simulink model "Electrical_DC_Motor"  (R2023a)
settings: Solver=VariableStepAuto  StartTime=0.0  StopTime=10.0  RelTol=1e-3
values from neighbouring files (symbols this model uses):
  K = 1    [Electrical_DC_Motor_EQN.m]    (also in Electrical_DC_Motor_SLX_m.m; SI_Units.m)
undefined symbols (not defined in the file or in its folder): eTr
libraries: fl_lib x8, nesl_utility x1

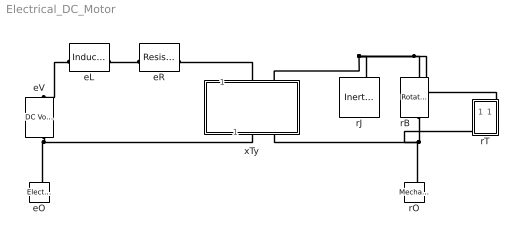
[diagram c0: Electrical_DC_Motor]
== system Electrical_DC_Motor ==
  eL : fl_lib/Electrical/Electrical Elements/Inductor  l=1e-6 H  r=0 Ohm  g=1e-9 1/Ohm  i_specify=off  i_priority=None  i=0 A  i_nominal_specify=off  i_nominal_unit=A  i_nominal_value=1  v_specify=off  v_priority=None  v=0 V  v_nominal_specify=off  v_nominal_unit=V  v_nominal_value=1  i_L_specify=off  i_L_priority=High  i_L=0 A  i_L_nominal_specify=off  i_L_nominal_unit=A  i_L_nominal_value=1
  eO : fl_lib/Electrical/Electrical Elements/Electrical Reference
  eR : fl_lib/Electrical/Electrical Elements/Resistor  R=1 Ohm  i_specify=off  i_priority=None  i=0 A  i_nominal_specify=off  i_nominal_unit=A  i_nominal_value=1  v_specify=off  v_priority=None  v=0 V  v_nominal_specify=off  v_nominal_unit=V  v_nominal_value=1
  eV : fl_lib/Electrical/Electrical Sources/DC Voltage Source  v0=1 V
  rB : fl_lib/Mechanical/Rotational Elements/Rotational Damper  D=0.001 N*m*s/rad  w_specify=off  w_priority=None  w=0 rad/s  w_nominal_specify=off  w_nominal_unit=rad/s  w_nominal_value=1  t_specify=off  t_priority=None  t=0 N*m  t_nominal_specify=off  t_nominal_unit=N*m  t_nominal_value=1
  rJ : fl_lib/Mechanical/Rotational Elements/Inertia  inertia=0.01 kg*m^2  num_ports=foundation.enum.numPorts2.one  w_specify=off  w_priority=High  w=0 rad/s  w_nominal_specify=off  w_nominal_unit=rad/s  w_nominal_value=1  t_specify=off  t_priority=None  t=0 N*m  t_nominal_specify=off  t_nominal_unit=N*m  t_nominal_value=1
  rO : fl_lib/Mechanical/Rotational Elements/Mechanical Rotational Reference
  rT : Subsystem  mask{rT='Ta'}
      mask prompts: rT "Output variable"
  xTy : Subsystem  mask{Transformer_type=eTr, T_type=F2=K*F1, xTy=K}
      mask prompts: Transformer_type "Type of Transformer"; T_type "Type of relation"; xTy "Name of parameter K"
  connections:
  eV/RConn1 -- xTy/RConn1 -- eO/LConn1
  eL/LConn1 -- eV/LConn1
  eR/LConn1 -- eL/RConn1
  xTy/LConn1 -- eR/RConn1
  rT/LConn1 -- rB/LConn1 -- xTy/LConn2 -- rJ/LConn1
  rB/RConn1 -- xTy/RConn2 -- rO/LConn1 -- rT/RConn1

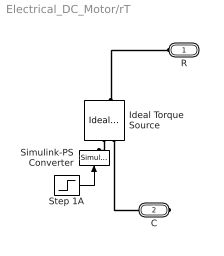
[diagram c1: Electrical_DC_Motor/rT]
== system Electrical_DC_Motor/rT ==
  Ideal Torque Source : fl_lib/Mechanical/Mechanical Sources/Ideal Torque Source
  Simulink-PS Converter : nesl_utility/Simulink-PS Converter  PhysicalDomain=network_engine_domain  SubClassName=ps_input  LeftPortType=input  RightPortType=output  PseudoPeriodic=off  Frequencies=[]  NoiseDistribution=none  NoiseParameters=[]  Unit=1  AffineConversion=off  FilteringAndDerivatives=zero  SimscapeFilterOrder=1  InputFilterTimeConstant=.001  UdotUserProvided=0
  Step 1A : Step  After=100  SampleTime=0
  R : PMIOPort  Side=Left
  C : PMIOPort  Port=2  Side=Right
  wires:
  Step 1A/1 -> Simulink-PS Converter/1
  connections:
  Ideal Torque Source/RConn2 -- C/RConn1
  Ideal Torque Source/LConn1 -- R/RConn1
  Ideal Torque Source/RConn1 -- Simulink-PS Converter/RConn1

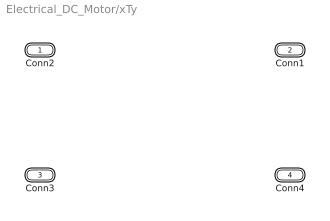
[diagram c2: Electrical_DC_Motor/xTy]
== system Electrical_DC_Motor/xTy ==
  Conn2 : PMIOPort  Side=Left
  Conn1 : PMIOPort  Port=2  Side=Left
  Conn3 : PMIOPort  Port=3  Side=Right
  Conn4 : PMIOPort  Port=4  Side=Right
